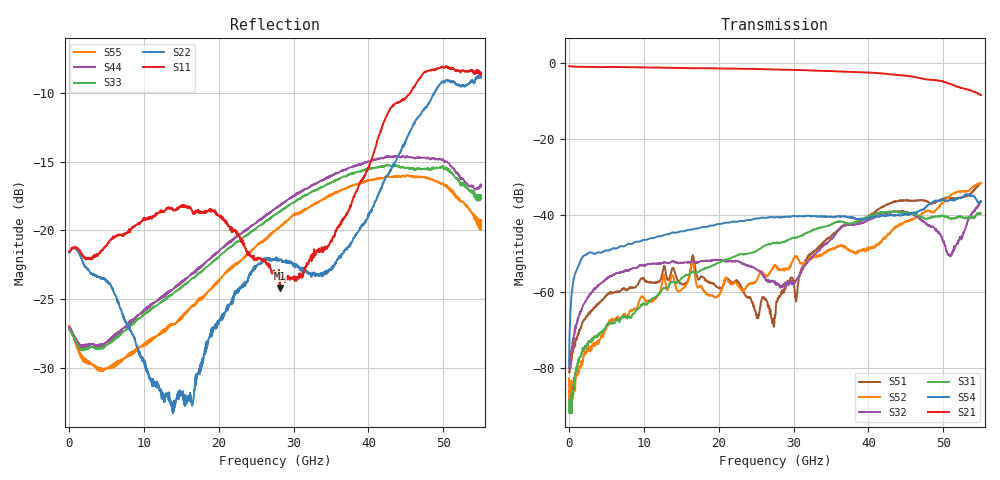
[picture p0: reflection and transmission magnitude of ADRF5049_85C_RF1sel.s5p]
! Device  : ADRF5049
! Description: Silicon SP4T Switch Non-Reflective
! Frequency:  9kHz -  45 GHz
! Ports:
!  RFC = Port 1
!  RF1 = Port 2
!  RF2 = Port 3
!	 RF3 = Port 4
!  RF4 = Port 5
! VSS  =  +3.30 Volts
! VDD  =  -3.30 Volts
! EN  =  0.00 Volts
! LS  =  0.00 Volts
! V1  =  0.00 Volts
! V2  =  0.00 Volts
! Data:  Data was collected using an calibrated 4 port network analyzer.
! Notes: Analog Devices supplies this data as a sample of measured data
!  for this product.  Your particular data for this product may vary.
!  Data was taken at 85C degrees C.
!  Analog Devices reserves the right to change this data at anytime.
# HZ S DB R 50
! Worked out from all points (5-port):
!   1100 points, 50 MHz to 55 GHz, reference 50 ohm
!   strongest paths, dB at 50 MHz, 13.8 GHz, 27.55 GHz, 41.3 GHz, 55 GHz:
!     S21: -0.8, -1.3, -1.7, -2.6, -8.4
!     S54: -79.4, -44.5, -40.5, -40.3, -36.4
!     S31: -88.6, -57.5, -47.2, -39.4, -39.5
!     S32: -80.0, -52.0, -57.4, -40.0, -36.3
!     S52: -82.8, -55.8, -53.0, -47.5, -31.5
!     S51: -81.1, -54.0, -66.5, -38.5, -31.4
!   lowest |S11| = -24.2 dB at 28.15 GHz (marker M1), VSWR 1.13, Z = 53.4 - j5.4 ohm
!   |S11| at or under -10 dB: start of sweep to 45.58 GHz
